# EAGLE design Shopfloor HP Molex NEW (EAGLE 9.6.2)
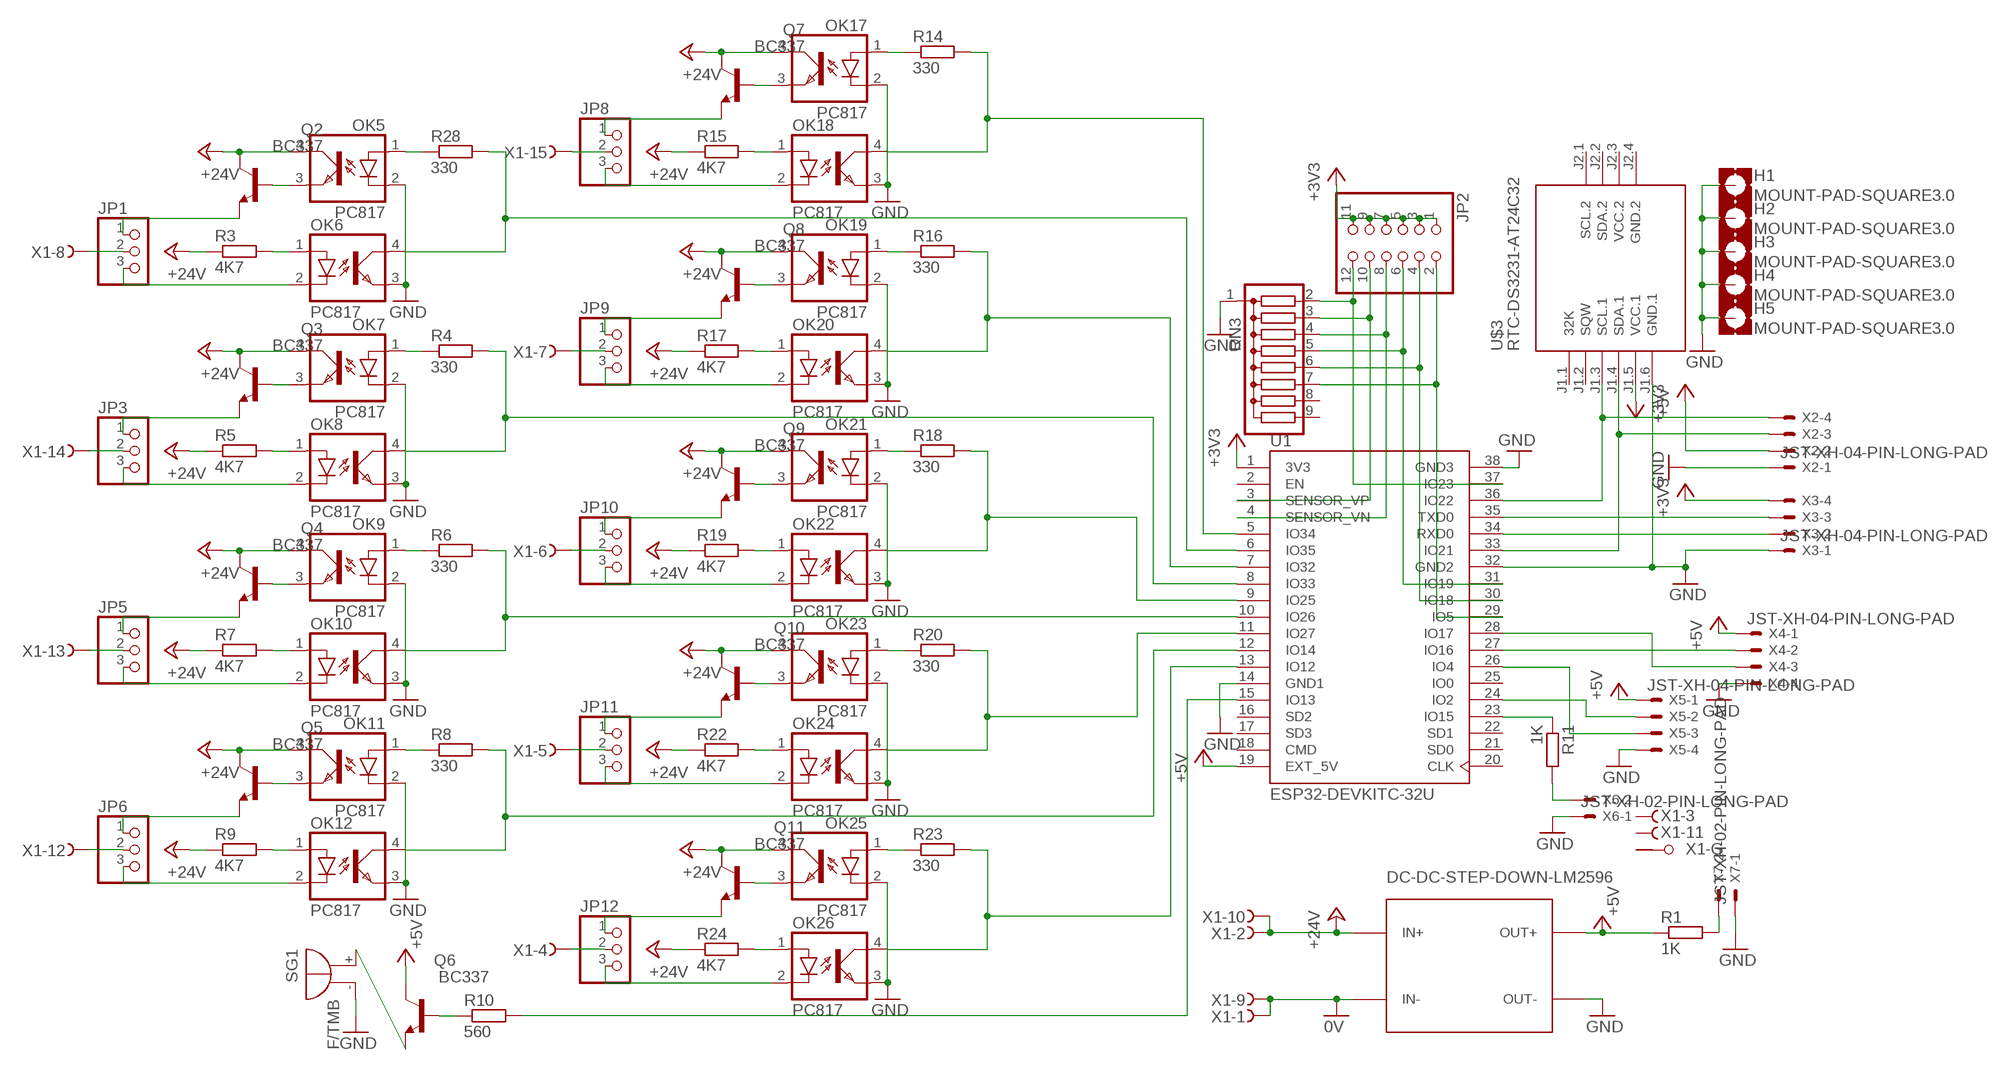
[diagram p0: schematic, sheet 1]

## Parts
H1  MOUNT-PAD-SQUARE3.0  [3,0-PAD-SQUARE]
H2  MOUNT-PAD-SQUARE3.0  [3,0-PAD-SQUARE]
H3  MOUNT-PAD-SQUARE3.0  [3,0-PAD-SQUARE]
H4  MOUNT-PAD-SQUARE3.0  [3,0-PAD-SQUARE]
H5  MOUNT-PAD-SQUARE3.0  [3,0-PAD-SQUARE]
JP1  PINHD-1X3  [1X03]
JP2  PINHD-2X6  [2X06]
JP3  PINHD-1X3  [1X03]
JP5  PINHD-1X3  [1X03]
JP6  PINHD-1X3  [1X03]
JP8  PINHD-1X3  [1X03]
JP9  PINHD-1X3  [1X03]
JP10  PINHD-1X3  [1X03]
JP11  PINHD-1X3  [1X03]
JP12  PINHD-1X3  [1X03]
OK5  PC817  [DIL04]
OK6  PC817  [DIL04]
OK7  PC817  [DIL04]
OK8  PC817  [DIL04]
OK9  PC817  [DIL04]
OK10  PC817  [DIL04]
OK11  PC817  [DIL04]
OK12  PC817  [DIL04]
OK17  PC817  [DIL04]
OK18  PC817  [DIL04]
OK19  PC817  [DIL04]
OK20  PC817  [DIL04]
OK21  PC817  [DIL04]
OK22  PC817  [DIL04]
OK23  PC817  [DIL04]
OK24  PC817  [DIL04]
OK25  PC817  [DIL04]
OK26  PC817  [DIL04]
Q2  BC337  [TO92]
Q3  BC337  [TO92]
Q4  BC337  [TO92]
Q5  BC337  [TO92]
Q6  BC337  [TO92]
Q7  BC337  [TO92]
Q8  BC337  [TO92]
Q9  BC337  [TO92]
Q10  BC337  [TO92]
Q11  BC337  [TO92]
R1  1K  R-EU_0207/7  [0207/7]
R3  4K7  R-EU_0207/7  [0207/7]
R4  330  R-EU_0207/7  [0207/7]
R5  4K7  R-EU_0207/7  [0207/7]
R6  330  R-EU_0207/7  [0207/7]
R7  4K7  R-EU_0207/7  [0207/7]
R8  330  R-EU_0207/7  [0207/7]
R9  4K7  R-EU_0207/7  [0207/7]
R10  560  R-EU_0207/7  [0207/7]
R11  1K  R-EU_0207/7  [0207/7]
R14  330  R-EU_0207/7  [0207/7]
R15  4K7  R-EU_0207/7  [0207/7]
R16  330  R-EU_0207/7  [0207/7]
R17  4K7  R-EU_0207/7  [0207/7]
R18  330  R-EU_0207/7  [0207/7]
R19  4K7  R-EU_0207/7  [0207/7]
R20  330  R-EU_0207/7  [0207/7]
R22  4K7  R-EU_0207/7  [0207/7]
R23  330  R-EU_0207/7  [0207/7]
R24  4K7  R-EU_0207/7  [0207/7]
R28  330  R-EU_0207/7  [0207/7]
RN3  G08R  [SIL9]
SG1  F/TMB  [F/TMB]
U1  ESP32-DEVKITC-32U  [MODULE_ESP32-DEVKITC-32U]
U$1  DC-DC-STEP-DOWN-LM2596  [DC-DC-STEP-DOWN-LM2596]
U$3  RTC-DS3231-AT24C32  [RTC-DS3231-AT24C32]
X1  F15HPS  [F15HP]
X2  JST-XH-04-PIN-LONG-PAD  [JST-XH-04-PACKAGE-LONG-PAD]
X3  JST-XH-04-PIN-LONG-PAD  [JST-XH-04-PACKAGE-LONG-PAD]
X4  JST-XH-04-PIN-LONG-PAD  [JST-XH-04-PACKAGE-LONG-PAD]
X5  JST-XH-04-PIN-LONG-PAD  [JST-XH-04-PACKAGE-LONG-PAD]
X6  JST-XH-02-PIN-LONG-PAD  [JST-XH-02-PACKAGE-LONG-PAD]
X7  JST-XH-02-PIN-LONG-PAD  [JST-XH-02-PACKAGE-LONG-PAD]

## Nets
0V: U$1.IN- X1.1(-1:F) X1.9(-9:F)
+3V3: JP2.1 JP2.3 JP2.5 JP2.7 JP2.9 JP2.11 U1.1(3V3) U$3.J1.5(VCC.1) X3.4
+5V: Q6.3(C) R1.1 U1.19(EXT_5V) U$1.OUT+ X2.2 X4.1 X5.1
+24V: OK5.4(COL) OK7.4(COL) OK9.4(COL) OK11.4(COL) OK17.4(COL) OK19.4(COL) OK21.4(COL) OK23.4(COL) OK25.4(COL) Q2.3(C) Q3.3(C) Q4.3(C) Q5.3(C) Q7.3(C) Q8.3(C) Q9.3(C) Q10.3(C) Q11.3(C) R3.1 R5.1 R7.1 R9.1 R15.1 R17.1 R19.1 R22.1 R24.1 U$1.IN+ X1.2(-2:F) X1.10(-10:F)
GND: H1.B3,0(MOUNT) H2.B3,0(MOUNT) H3.B3,0(MOUNT) H4.B3,0(MOUNT) H5.B3,0(MOUNT) OK5.2(C) OK6.3(EMIT) OK7.2(C) OK8.3(EMIT) OK9.2(C) OK10.3(EMIT) OK11.2(C) OK12.3(EMIT) OK17.2(C) OK18.3(EMIT) OK19.2(C) OK20.3(EMIT) OK21.2(C) OK22.3(EMIT) OK23.2(C) OK24.3(EMIT) OK25.2(C) OK26.3(EMIT) RN3.1 SG1.- U1.14(GND1) U1.32(GND2) U1.38(GND3) U$1.OUT- U$3.J1.6(GND.1) X2.1 X3.1 X4.4 X5.4 X6.1 X7.1
N$1: U1.35(TXD0) X3.3
N$2: JP2.12 RN3.2 U1.37(IO23)
N$3: R11.2 X6.2
N$4: JP1.2 X1.8(-8:F)
N$5: U1.27(IO16) X4.2
N$6: JP2.10 RN3.3 U1.3(SENSOR_VP)
N$7: JP2.8 RN3.4 U1.4(SENSOR_VN)
N$8: JP2.6 RN3.5 U1.31(IO19)
N$9: U1.26(IO4) X5.3
N$10: U1.24(IO2) X5.2
N$11: R11.1 U1.23(IO15)
N$12: Q6.2(B) R10.1
N$13: JP2.4 RN3.6 U1.30(IO18)
N$14: Q6.1(E) SG1.+
N$15: JP8.2 X1.15(-15:F)
N$16: R1.2 X7.2
N$17: JP2.2 RN3.7 U1.29(IO5)
N$19: OK6.4(COL) R28.2 U1.6(IO35)
N$20: OK20.4(COL) R16.2 U1.7(IO32)
N$21: OK8.4(COL) R4.2 U1.8(IO33)
N$22: OK22.4(COL) R18.2 U1.9(IO25)
N$23: OK10.4(COL) R6.2 U1.10(IO26)
N$24: OK24.4(COL) R20.2 U1.11(IO27)
N$25: U1.28(IO17) X4.3
N$26: OK12.4(COL) R8.2 U1.12(IO14)
N$27: U1.33(IO21) U$3.J1.4(SDA.1) X2.3
N$28: OK26.4(COL) R23.2 U1.13(IO12)
N$29: U1.36(IO22) U$3.J1.3(SCL.1) X2.4
N$30: R10.2 U1.15(IO13)
N$31: OK5.1(A) R28.1
N$32: OK5.3(EMIT) Q2.2(B)
N$33: OK6.1(A) R3.2
N$34: JP1.1 Q2.1(E)
N$35: JP1.3 OK6.2(C)
N$36: JP9.2 X1.7(-7:F)
N$37: OK7.1(A) R4.1
N$38: OK7.3(EMIT) Q3.2(B)
N$39: OK8.1(A) R5.2
N$40: JP3.1 Q3.1(E)
N$41: JP3.3 OK8.2(C)
N$42: JP10.2 X1.6(-6:F)
N$43: OK9.1(A) R6.1
N$44: OK9.3(EMIT) Q4.2(B)
N$45: OK10.1(A) R7.2
N$46: U1.34(RXD0) X3.2
N$47: JP5.1 Q4.1(E)
N$48: JP5.3 OK10.2(C)
N$49: JP11.2 X1.5(-5:F)
N$50: OK11.1(A) R8.1
N$51: OK11.3(EMIT) Q5.2(B)
N$52: OK12.1(A) R9.2
N$53: JP6.1 Q5.1(E)
N$54: JP6.3 OK12.2(C)
N$55: OK18.4(COL) R14.2 U1.5(IO34)
N$56: JP12.2 X1.4(-4:F)
N$63: OK17.1(A) R14.1
N$64: OK17.3(EMIT) Q7.2(B)
N$65: OK18.1(A) R15.2
N$66: JP8.1 Q7.1(E)
N$68: JP8.3 OK18.2(C)
N$69: JP6.2 X1.12(-12:F)
N$70: OK19.1(A) R16.1
N$71: OK19.3(EMIT) Q8.2(B)
N$72: OK20.1(A) R17.2
N$73: JP9.1 Q8.1(E)
N$74: JP9.3 OK20.2(C)
N$75: JP5.2 X1.13(-13:F)
N$76: OK21.1(A) R18.1
N$77: OK21.3(EMIT) Q9.2(B)
N$78: OK22.1(A) R19.2
N$79: JP10.1 Q9.1(E)
N$80: JP10.3 OK22.2(C)
N$81: JP3.2 X1.14(-14:F)
N$82: OK23.1(A) R20.1
N$83: OK23.3(EMIT) Q10.2(B)
N$84: OK24.1(A) R22.2
N$85: JP11.1 Q10.1(E)
N$86: JP11.3 OK24.2(C)
N$88: OK25.1(A) R23.1
N$89: OK25.3(EMIT) Q11.2(B)
N$90: OK26.1(A) R24.2
N$91: JP12.1 Q11.1(E)
N$92: JP12.3 OK26.2(C)
Unconnected: RN3.8 RN3.9 U1.2(EN) U1.16(SD2) U1.17(SD3) U1.18(CMD) U1.20(CLK) U1.21(SD0) U1.22(SD1) U1.25(IO0) U$3.J1.1(32K) U$3.J1.2(SQW) U$3.J2.1(SCL.2) U$3.J2.2(SDA.2) X1.3(-3:F) X1.11(-11:F) X1.G1(-G:G1) X1.G2(-G:G2)

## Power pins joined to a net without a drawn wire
GND.2: U$3.J2.4(GND.2)
VCC.2: U$3.J2.3(VCC.2)

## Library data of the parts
H1-H5 = holes:MOUNT-PAD-SQUARE: MOUNTING PAD, square
JP1 JP3 JP5 JP6 JP8-JP12 = pinhead:PINHD-1X3: PIN HEADER
JP2 = pinhead:PINHD-2X6: PIN HEADER
OK5-OK12 OK17-OK26 = optocoupler:PC817: SHARP OPTO COUPLER; MPN: PC817X4J000F; OC_FARNELL: 9707727; OC_NEWARK: 97K7059
Q2-Q11 = transistor-npn:BC337*: NPN Transistor
R1 R3-R11 R14-R20 R22-R24 R28 = rcl:R-EU_: RESISTOR, European symbol; SPICEPREFIX: R
RN3 = resistor-sil:G08R: SIL RESISTOR; OC_FARNELL: unknown; OC_NEWARK: unknown
SG1 = buzzer:F/TMB: BUZZER; OC_FARNELL: unknown; OC_NEWARK: unknown
U1 = ESP32-DEVKITC-32U:ESP32-DEVKITC-32U: ESP32-DEVKITC Check prices; AVAILABILITY: In Stock; DESCRIPTION: ESP32-WROOM-32UE - Transceiver; 802.11 b/g/n (Wi-Fi, WiFi, WLAN), Bluetooth® Smart Ready 4.x Dual Mode Evaluation Board; MF: Espressif Systems; MP: ESP32-DEVKITC-32U; PACKAGE: None; PRICE: None
U$1 = diy-modules:DC-DC-STEP-DOWN-LM2596: DC/DC Step-Down Regulator based on LM2596-ADJ chip LM2596 datasheet available here: http://www.ti.com/lit/ds/symlink/lm2596.pdf Click here to find device on ebay.com
U$3 = diy-modules-ori:RTC-DS3231-AT24C32: RTC Module with Battery and EEPROM based on DS3231 and AT24C32 chips Tutorial can be found here: https://edwardmallon.wordpress.com/2014/05/21/using-a-cheap-3-ds3231-rtc-at24c32-eeprom-from-ebay/ Click here to find device on ebay.com
X1 = con-subd:F15HPS: SUB-D; OC_FARNELL: unknown; OC_NEWARK: unknown
X2-X5 = Rembrandt Electronics - JST XH Connectors v1-0:JST-XH-04-PIN: JST XH Connector 2 Pin Wire to board connector. Pitch: 2,54 mm, (0.100") Number of pins: 4 Created by Rembrandt Electronics www.rembrandtelectronics.com
X6 X7 = Rembrandt Electronics - JST XH Connectors v1-0:JST-XH-02-PIN: JST XH Connector 2 Pin

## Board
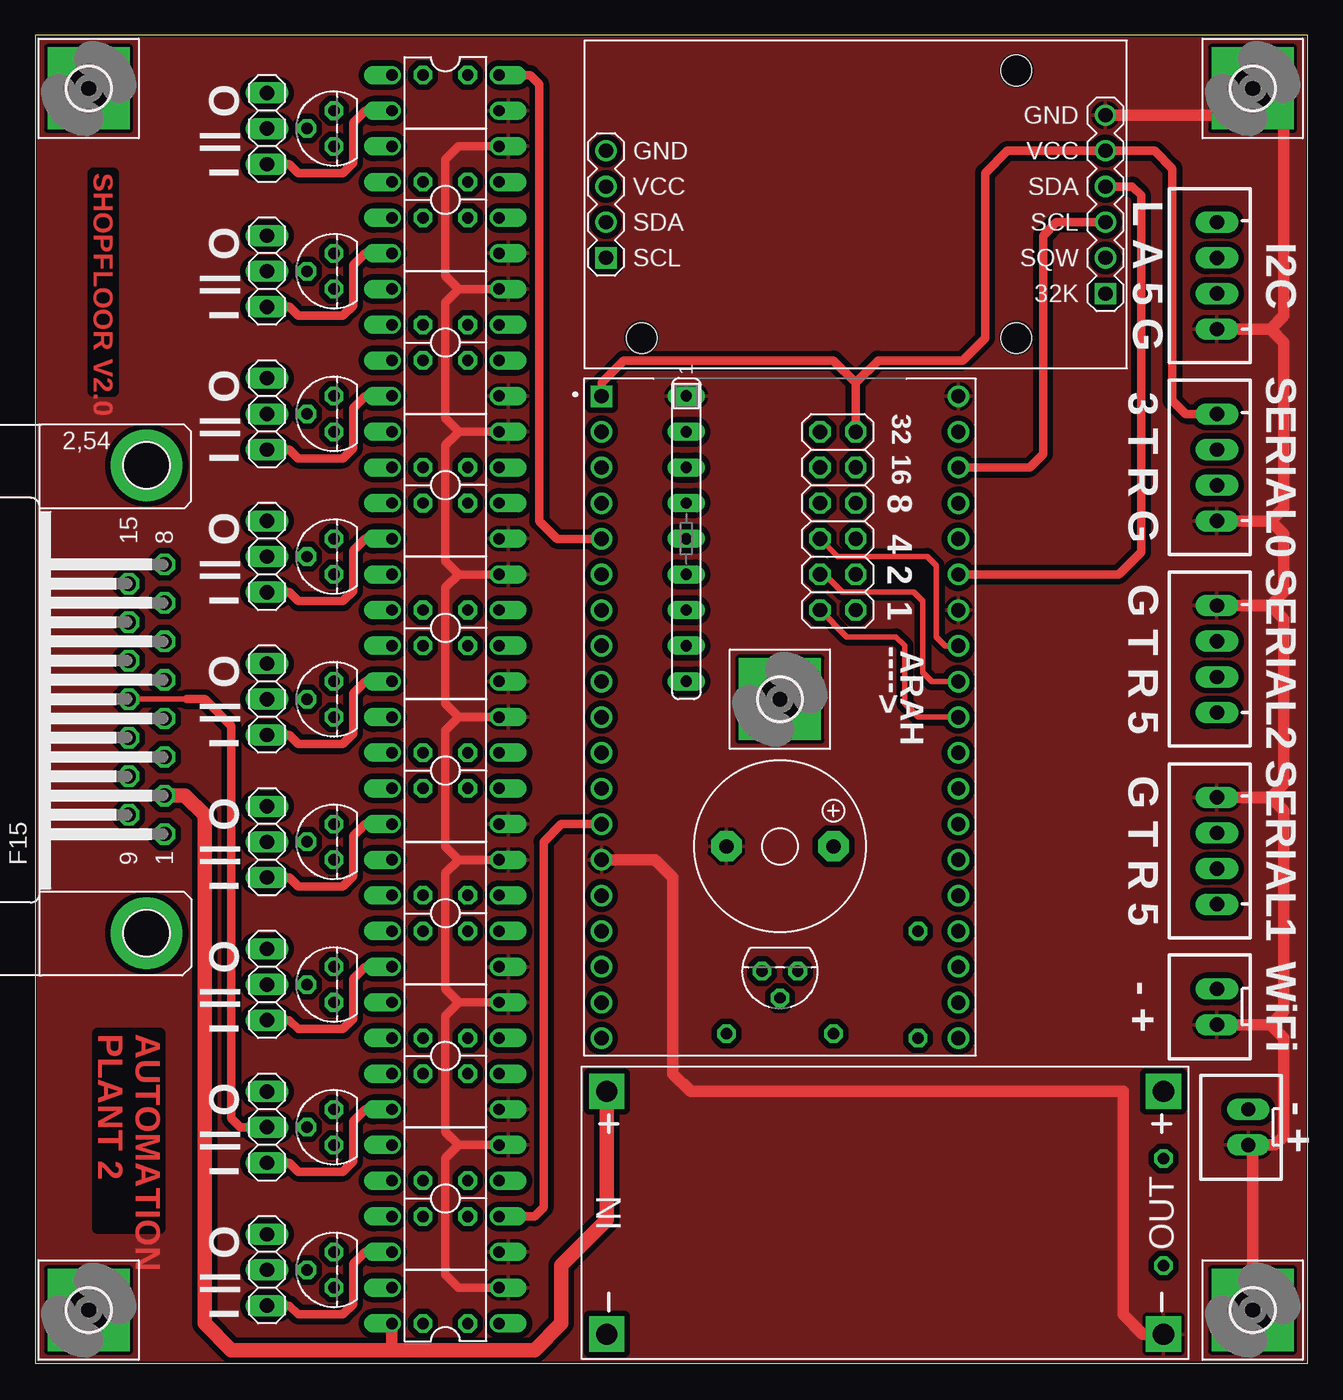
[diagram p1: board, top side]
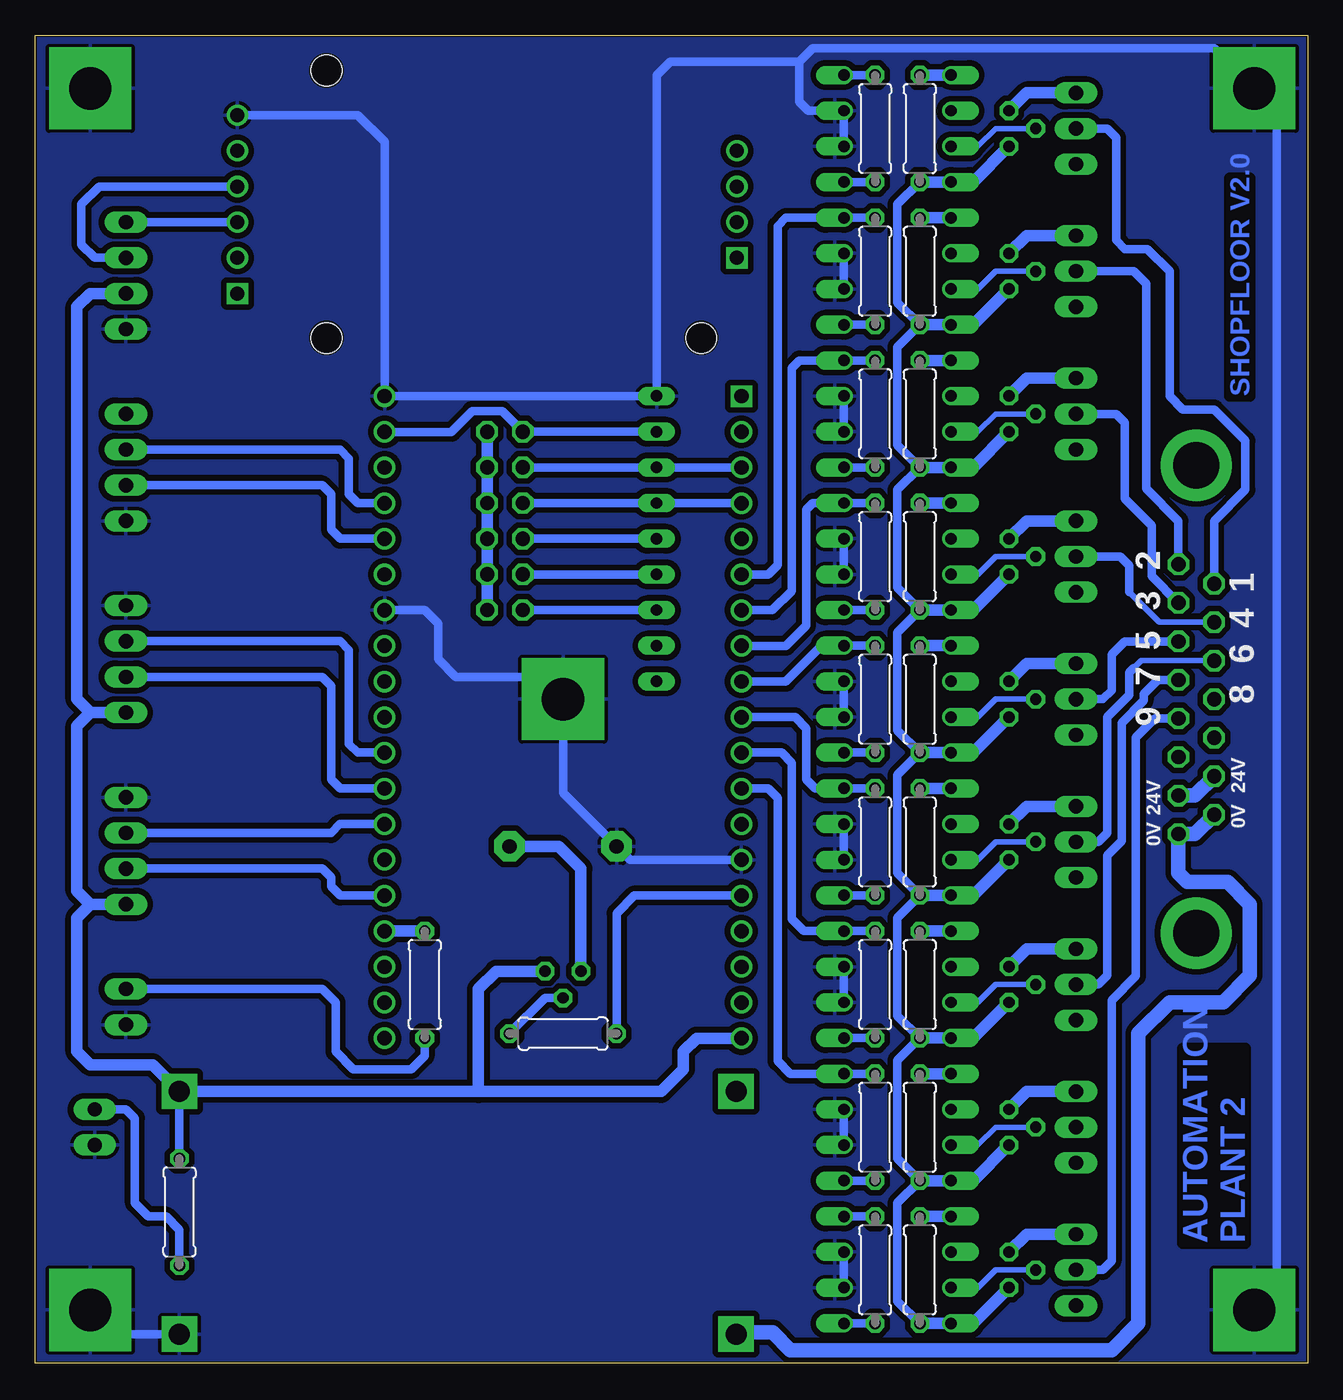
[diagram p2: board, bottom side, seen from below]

Size 90.6 x 94.6 mm. Coordinates in mm from the lower left corner, seen from the top.
Outline: 0,0 90.6,0 90.6,94.6 0,94.6 0,0
Copper layers (1*16): Top 0.035mm / dielectric 1.5mm / Bottom 0.035mm
Design rules "default *": minimum track width 6mil, minimum drill 0.35mm, track to track 16mil, track to pad 16mil, pad to pad 16mil, via to via 16mil, smd to smd 18mil, copper to edge 5mil, drill to drill 6mil, minimum pad ring 10mil, minimum via ring 8mil, stop-mask expansion 4mil, vias tented up to drill 0mil, thermal gap 10mil

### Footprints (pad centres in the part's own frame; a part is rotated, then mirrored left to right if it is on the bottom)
3,0-PAD-SQUARE = drill 3 pad 5.842 square: B3,0 0,0
1X03 = drill 1.016 long: 1 -2.54,0; 2 0,0; 3 2.54,0
2X06 = drill 1.016 octagon: 1 -6.35,-1.27; 2 -6.35,1.27; 3 -3.81,-1.27; 4 -3.81,1.27; 5 -1.27,-1.27; 6 -1.27,1.27; 7 1.27,-1.27; 8 1.27,1.27; 9 3.81,-1.27; 10 3.81,1.27; 11 6.35,-1.27; 12 6.35,1.27
DIL04 = drill 0.813 offset: 1 -1.27,-3.81; 2 1.27,-3.81; 3 1.27,3.81; 4 -1.27,3.81
TO92 = drill 0.813 octagon: 1 1.27,0; 2 0,1.905; 3 -1.27,0
0207/7 = drill 0.813 octagon: 1 -3.81,0; 2 3.81,0
SIL9 = drill 0.813 long: 1 -10.16,0; 2 -7.62,0; 3 -5.08,0; 4 -2.54,0; 5 0,0; 6 2.54,0; 7 5.08,0; 8 7.62,0; 9 10.16,0
F/TMB = drill 1.016 pad 2.159 octagon: + 3.81,0; - -3.81,0
MODULE_ESP32-DEVKITC-32U = drill 1.02 square: 1 -12.7,22.85 | drill 1.02: 2 -12.7,20.31; 3 -12.7,17.77; 4 -12.7,15.23; 5 -12.7,12.69; 6 -12.7,10.15; 7 -12.7,7.61; 8 -12.7,5.07; 9 -12.7,2.53; 10 -12.7,-0.01; 11 -12.7,-2.55; 12 -12.7,-5.09; 13 -12.7,-7.63; 14 -12.7,-10.17; 15 -12.7,-12.71; 16 -12.7,-15.25; 17 -12.7,-17.79; 18 -12.7,-20.33; 19 -12.7,-22.87; 20 12.7,-22.87; 21 12.7,-20.33; 22 12.7,-17.79; 23 12.7,-15.25; 24 12.7,-12.71; 25 12.7,-10.17; 26 12.7,-7.63; 27 12.7,-5.09; 28 12.7,-2.55; 29 12.7,-0.01; 30 12.7,2.53; 31 12.7,5.07; 32 12.7,7.61; 33 12.7,10.15; 34 12.7,12.69; 35 12.7,15.23; 36 12.7,17.77; 37 12.7,20.31; 38 12.7,22.85
DC-DC-STEP-DOWN-LM2596 = drill 1.5 pad 2.5 square: IN+ -19.812,8.636; IN- -19.812,-8.636; OUT+ 19.812,8.636; OUT- 19.812,-8.636
RTC-DS3231-AT24C32 = drill 1 square: J1.1 -17.78,6.35; J2.1 17.78,3.81 | drill 1: J1.2 -17.78,3.81; J1.3 -17.78,1.27; J1.4 -17.78,-1.27; J1.5 -17.78,-3.81; J1.6 -17.78,-6.35; J2.2 17.78,1.27; J2.3 17.78,-1.27; J2.4 17.78,-3.81 | hole 2.2: -11.43,-9.525; -11.43,9.525; 15.24,9.525
F15HP = drill 1.016 octagon: 1 -9.601,-1.27; 2 -6.858,-1.27; 3 -4.115,-1.27; 4 -1.372,-1.27; 5 1.372,-1.27; 6 4.115,-1.27; 7 6.858,-1.27; 8 9.601,-1.27; 9 -8.23,1.27; 10 -5.486,1.27; 11 -2.743,1.27; 12 0,1.27; 13 2.743,1.27; 14 5.486,1.27; 15 8.23,1.27 | drill 3.302 pad 5.08: G1 -16.662,0; G2 16.662,0
JST-XH-04-PACKAGE-LONG-PAD = drill 1.016 long: 1 -3.81,0; 2 -1.27,0; 3 1.27,0; 4 3.81,0
JST-XH-02-PACKAGE-LONG-PAD = drill 1.016 long: 1 -1.27,0; 2 1.27,0

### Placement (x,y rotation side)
H1  3.81,3.81 0 top
H2  3.81,90.81 0 top
H3  53.02,47.31 0 top
H4  86.68,3.81 0 top
H5  86.68,90.81 0 top
JP1  16.51,77.79 270 top
JP2  57.15,60.01 90 top
JP3  16.51,57.47 270 top
JP5  16.51,37.15 270 top
JP6  16.51,16.83 270 top
JP8  16.51,87.95 270 top
JP9  16.51,67.63 270 top
JP10  16.51,47.31 270 top
JP11  16.51,26.99 270 top
JP12  16.51,6.67 270 top
OK5  29.21,75.25 90 top
OK6  29.21,80.33 270 top
OK7  29.21,54.93 90 top
OK8  29.21,60.01 270 top
OK9  29.21,34.61 90 top
OK10  29.21,39.69 270 top
OK11  29.21,14.29 90 top
OK12  29.21,19.37 270 top
OK17  29.21,85.41 90 top
OK18  29.21,90.49 270 top
OK19  29.21,65.09 90 top
OK20  29.21,70.17 270 top
OK21  29.21,44.77 90 top
OK22  29.21,49.85 270 top
OK23  29.21,24.45 90 top
OK24  29.21,29.53 270 top
OK25  29.21,4.13 90 top
OK26  29.21,9.21 270 top
Q2  21.27,77.79 90 top
Q3  21.27,57.47 90 top
Q4  21.27,37.15 90 top
Q5  21.27,16.83 90 top
Q6  53.02,27.94 180 top
Q7  21.27,87.95 90 top
Q8  21.27,67.63 90 top
Q9  21.27,47.31 90 top
Q10  21.27,26.99 90 top
Q11  21.27,6.67 90 top
R1  80.33,10.79 270 bottom
R3  27.62,77.79 90 bottom
R4  30.8,57.47 90 bottom
R5  27.62,57.47 90 bottom
R6  30.8,37.15 90 bottom
R7  27.62,37.15 90 bottom
R8  30.8,16.83 90 bottom
R9  27.62,16.83 90 bottom
R10  53.02,23.5 0 bottom
R11  62.87,26.99 270 bottom
R14  30.8,87.95 90 bottom
R15  27.62,87.95 90 bottom
R16  30.8,67.63 90 bottom
R17  27.62,67.63 90 bottom
R18  30.8,47.31 90 bottom
R19  27.62,47.31 90 bottom
R20  30.8,26.99 90 bottom
R22  27.62,26.99 90 bottom
R23  30.8,6.67 90 bottom
R24  27.62,6.67 90 bottom
R28  30.8,77.79 90 bottom
RN3  46.35,58.74 270 top
SG1  53.02,36.83 0 top
U1  53.02,46.04 0 top
U$1  60.52,10.73 0 top
U$3  58.42,82.55 180 top
X1  7.94,47.31 90 top
X2  84.14,77.47 90 top
X3  84.14,63.82 90 top
X4  84.14,50.16 90 top
X5  84.14,36.51 90 top
X6  84.14,25.4 90 top
X7  86.36,16.83 90 top

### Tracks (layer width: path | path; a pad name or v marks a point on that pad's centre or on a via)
0V
  Bottom 1.016: X1.9 8.04,37.71 X1.1 9.21,34.92 8.57,34.29 5.71,34.29 4.13,32.7 4.13,27.62 6.03,25.72 9.84,25.72 12.06,23.5 12.06,2.86 13.97,0.95 36.83,0.95 38.1,2.22 40.58,2.22 U$1.IN-
+3V3
  Top 0.61: U1.1 40.32,69.85 41.91,71.44 56.83,71.44 58.42,69.85 | JP2.11 58.42,69.85 | 58.42,69.85 60.01,71.44 66.04,71.44 67.63,73.03 67.63,84.77 69.22,86.36 U$3.J1.5 79.69,86.36 80.96,85.09 80.96,68.58 81.92,67.63 X3.4
  Bottom 0.813: JP2.11 JP2.9 JP2.7 JP2.5 JP2.3 JP2.1
+5V
  Bottom 0.61: U$1.OUT+ R1.1
  Bottom 0.813: U1.19 43.51,23.17 44.45,22.23 44.45,20.95 46.04,19.37 59.05,19.37 | 59.05,19.37 U$1.OUT+ 82.23,21.27 86.68,21.27 87.63,22.23 87.63,31.75 86.68,32.7 | Q6.3 57.78,27.94 59.05,26.67 59.05,19.37 | X5.1 86.68,32.7 | 86.68,32.7 87.63,33.66 87.63,45.4 86.68,46.35 | X4.1 86.68,46.35 | 86.68,46.35 87.63,47.31 87.63,75.25 86.68,76.2 X2.2
+24V
  Top 0.813: OK25.4 25.4,0.95
  Top 1.016: X1.2 10.67,40.45 12.06,39.05 12.06,2.86 13.97,0.95 25.4,0.95 35.56,0.95 37.47,2.86 37.47,6.99 40.7,10.22 U$1.IN+
  Bottom 0.61: R15.1 29.21,82.55 29.21,75.56 R3.1 29.21,72.39 29.21,65.41 R17.1 29.21,62.23 29.21,55.24 R5.1 29.21,52.07 29.21,45.09 R19.1 29.21,41.91 29.21,34.92 R7.1 29.21,31.75 29.21,24.77 R22.1 29.21,21.59 29.21,14.61 R9.1 29.21,11.43 29.21,4.45 R24.1
  Bottom 0.813: R24.1 OK25.4 23.81,2.86 Q11.3 | R9.1 OK11.4 23.81,13.02 Q5.3 | R22.1 OK23.4 23.81,23.18 Q10.3 | R7.1 OK9.4 23.81,33.34 Q4.3 | R19.1 OK21.4 23.81,43.5 Q9.3 | R5.1 OK7.4 23.81,53.66 Q3.3 | R17.1 OK19.4 23.81,63.82 Q8.3 | R3.1 OK5.4 23.81,73.98 Q2.3 | R15.1 OK17.4 23.81,84.14 Q7.3
  Bottom 1.016: X1.10 8.04,40.45 X1.2
GND
  Top 0.61: OK17.2 30.16,86.68 29.21,85.72 29.21,77.47 30.16,76.52 | OK5.2 30.16,76.52 | 30.16,76.52 29.21,75.56 29.21,67.31 30,66.52 | 30,66.52 30.16,66.36 OK19.2 | 30,66.52 30,66.2 29.21,65.41 29.21,57.15 30.16,56.2 | OK7.2 30.16,56.2 | 30.16,56.2 29.21,55.24 29.21,46.99 30.16,46.04 | OK21.2 30.16,46.04 | 30.16,46.04 29.21,45.09 29.21,36.83 30.16,35.88 | OK9.2 30.16,35.88 | 30.16,35.88 29.21,34.92 29.21,26.67 30.16,25.72 | OK23.2 30.16,25.72 | 30.16,25.72 29.21,24.77 29.21,16.51 30.16,15.56 | OK11.2 30.16,15.56 | 30.16,15.56 29.21,14.61 29.21,6.35 30.16,5.4 OK25.2
  Top 0.813: U$1.OUT- 78.87,2.1 77.47,3.49 77.47,19.37 46.67,19.37 45.4,20.64 45.4,34.61 44.14,35.87 U1.14 | H4.B3,0 86.68,15.24 X7.1 88.27,15.56 88.9,16.19 88.9,23.18 87.95,24.13 | 87.95,24.13 X6.1 | 87.95,24.13 88.9,25.08 88.9,39.37 87.95,40.32 | 87.95,53.98 88.9,53.02 88.9,41.27 87.95,40.32 | X4.4 87.95,53.98 | 87.95,53.98 88.9,54.93 88.9,59.05 87.95,60.01 | X3.1 87.95,60.01 | 87.95,60.01 88.9,60.96 88.9,72.71 87.95,73.66 | X2.1 87.95,73.66 | 87.95,73.66 88.9,74.61 88.9,89.53 87.63,90.81 H5.B3,0 84.77,88.9 U$3.J1.6 | 87.95,40.32 X5.4
  Bottom 0.61: U1.14 48.25,35.87 SG1.- 53.02,40.64 H3.B3,0 54.61,48.9 60.64,48.9 61.91,50.16 61.91,52.7 62.87,53.66 U1.32 | U$3.J1.6 67.63,88.9 65.72,87 U1.38 RN3.1 46.35,91.76 45.4,92.71 36.2,92.71 | H1.B3,0 2.22,5.4 2.22,89.22 H2.B3,0 6.67,93.66 35.24,93.66 36.2,92.71 | OK26.3 OK25.2 | OK11.2 OK12.3 | OK23.2 OK24.3 | OK10.3 OK9.2 | OK22.3 OK21.2 | OK7.2 OK8.3 | OK20.3 OK19.2 | OK17.2 OK18.3 35.56,89.22 36.2,89.85 36.2,92.71 | OK6.3 OK5.2 | U$1.OUT- 84.96,2.1 H4.B3,0
  pour Top: 0,94.61 90.49,94.61 90.49,94.3 90.49,0 89.85,0 0,0
  pour Bottom: 0,94.61 90.49,94.61 90.49,94.3 90.49,0 90.17,0 0,0
N$1
  Bottom 0.61: 65.73,61.28 U1.35 67.62,61.27 68.26,61.91 68.26,64.45 68.9,65.09 X3.3
N$2
  Bottom 0.61: RN3.2 JP2.12 57.35,67.83 59.49,67.83 60.97,66.35 U1.37
N$3
  Bottom 0.61: R11.2 62.87,21.91 63.82,20.95 67.94,20.95 69.22,22.23 69.22,25.72 70.17,26.67 X6.2
N$4
  Bottom 0.61: X1.8 9.21,60.01 11.51,62.31 11.51,76.91 12.38,77.79 JP1.2
N$5
  Bottom 0.61: U1.27 65.73,40.96 68.9,40.96 69.53,41.59 69.53,48.26 70.17,48.9 X4.2
N$6
  Bottom 0.61: JP2.10 RN3.3 46.34,63.81 U1.3
N$7
  Bottom 0.61: U1.4 40.33,61.28 RN3.4 JP2.8
N$8
  Top 0.406: JP2.6 57.15,57.47 63.5,57.47 64.14,56.83 64.14,51.75 64.78,51.11 U1.31
  Bottom 0.61: RN3.5 JP2.6
N$9
  Bottom 0.61: U1.26 68.91,38.41 69.53,37.78 X5.3
N$10
  Bottom 0.61: U1.24 68.89,33.33 69.53,33.97 69.53,34.61 70.17,35.24 X5.2
N$11
  Bottom 0.813: R11.1 U1.23
N$12
  Bottom 0.61: Q6.2 54.29,26.04 R10.1
N$13
  Top 0.406: JP2.4 56.2,56.2 57.47,54.93 62.55,54.93 63.18,54.29 63.18,49.21 63.83,48.57 U1.30
  Bottom 0.61: JP2.4 RN3.6
N$14
  Bottom 0.813: Q6.1 51.75,35.24 53.34,36.83 SG1.+
N$15
  Bottom 0.61: X1.15 6.67,60.01 4.45,62.23 4.45,65.72 6.67,67.94 8.89,67.94 9.84,68.9 9.84,77.79 11.43,79.38 13.02,79.38 13.65,80.01 13.65,87.31 14.29,87.95 JP8.2
N$16
  Bottom 0.61: R1.2 80.33,9.53 81.28,10.48 82.55,10.48 83.5,11.43 83.5,17.46 84.14,18.1 X7.2
N$17
  Top 0.406: JP2.2 57.78,51.75 61.28,51.75 61.91,51.12 61.91,46.99 62.88,46.03 U1.29
  Bottom 0.61: RN3.7 JP2.2
N$19
  Bottom 0.61: U1.6 38.43,56.19 37.74,56.87 37.74,81 37.15,81.6 OK6.4 R28.2
N$20
  Bottom 0.61: U1.7 38.11,53.65 36.73,55.03 36.73,70.9 36.2,71.44 OK20.4 R16.2
N$21
  Bottom 0.61: U1.8 37.16,51.11 35.71,52.55 35.71,60.81 35.24,61.28 OK8.4 R4.2
N$22
  Bottom 0.61: U1.9 37.16,48.57 34.61,51.12 OK22.4 R18.2
N$23
  Bottom 0.61: U1.10 36.5,46.03 35.71,45.24 35.71,41.59 35.08,40.96 OK10.4 R6.2
N$24
  Bottom 0.61: U1.11 37.47,43.5 36.73,42.76 36.73,31.65 35.88,30.8 OK24.4 R20.2
N$25
  Bottom 0.61: U1.28 65.73,43.5 67.63,43.5 68.26,44.13 68.26,50.8 68.9,51.44 X4.3
N$26
  Bottom 0.61: U1.12 38.42,40.96 37.74,40.28 37.74,21.55 36.83,20.64 OK12.4 R8.2
N$27
  Top 0.61: U1.33 77.14,56.19 78.74,57.78 78.74,83.19 78.11,83.82 U$3.J1.4
  Bottom 0.61: U$3.J1.4 86.04,83.82 87.31,82.55 87.31,79.69 86.36,78.74 X2.3
N$28
  Top 0.61: U1.13 37.45,38.41 36.2,37.15 36.2,11.11 35.56,10.48 OK26.4
  Bottom 0.61: R23.2 OK26.4
N$29
  Top 0.61: U1.36 70.79,63.81 71.75,64.77 71.75,80.33 72.71,81.28 U$3.J1.3
  Bottom 0.61: U$3.J1.3 X2.4
N$30
  Bottom 0.61: U1.15 47.95,33.33 49.21,32.07 R10.2
N$31
  Bottom 0.61: R28.1 OK5.1
N$32
  Bottom 0.406: Q2.2 22.23,77.79 23.5,76.52 OK5.3
N$33
  Bottom 0.813: R3.2 OK6.1
N$34
  Bottom 0.813: JP1.1 20,80.33 Q2.1
N$35
  Top 0.61: JP1.3 18.1,75.25 18.73,74.61 21.91,74.61 22.64,75.35 22.64,78.21 23.5,79.06 OK6.2
N$36
  Bottom 0.61: X1.7 11.11,56.07 11.11,59.69 13.02,61.59 13.02,66.99 13.65,67.63 JP9.2
N$37
  Bottom 0.61: R4.1 OK7.1
N$38
  Bottom 0.406: Q3.2 22.23,57.47 23.5,56.2 OK7.3
N$39
  Bottom 0.813: R5.2 OK8.1
N$40
  Bottom 0.813: JP3.1 20,60.01 Q3.1
N$41
  Top 0.61: JP3.3 18.1,54.93 18.73,54.29 21.91,54.29 22.64,55.03 22.64,57.89 23.5,58.74 OK8.2
N$42
  Bottom 0.61: X1.6 13.03,51.42 13.97,50.48 13.97,47.94 14.61,47.31 JP10.2
N$43
  Bottom 0.61: R6.1 OK9.1
N$44
  Bottom 0.406: Q4.2 22.23,37.15 23.5,35.88 OK9.3
N$45
  Bottom 0.813: R7.2 OK10.1
N$46
  Bottom 0.61: U1.34 65.73,58.74 68.9,58.74 69.53,59.37 69.53,61.91 70.17,62.55 X3.2
N$47
  Bottom 0.813: JP5.1 20,39.69 Q4.1
N$48
  Top 0.61: JP5.3 18.1,34.61 18.73,33.97 21.91,33.97 22.64,34.71 22.64,37.57 23.5,38.42 OK10.2
N$49
  Bottom 0.61: X1.5 10.69,48.68 11.68,47.69 11.68,47.2 13.26,45.63 13.26,37.22 14.29,36.2 14.29,35.23 14.28,35.22 14.28,28.92 14.29,28.91 14.29,27.62 14.92,26.99 JP11.2
N$50
  Bottom 0.61: R8.1 OK11.1
N$51
  Bottom 0.406: Q5.2 22.23,16.83 23.5,15.56 OK11.3
N$52
  Bottom 0.813: R9.2 OK12.1
N$53
  Bottom 0.813: JP6.1 20,19.37 Q5.1
N$54
  Top 0.61: JP6.3 18.1,14.29 18.73,13.65 21.91,13.65 22.64,14.39 22.64,17.25 23.5,18.1 OK12.2
N$55
  Top 0.61: U1.5 37.16,58.73 35.88,60.01 35.88,87.31 35.88,88.58 35.88,91.12 35.24,91.76 OK18.4
  Bottom 0.61: R14.2 OK18.4
N$56
  Bottom 0.61: X1.4 10.9,45.94 12.24,44.59 12.24,27.59 13.97,25.87 13.97,7.3 14.61,6.67 JP12.2
N$63
  Bottom 0.61: R14.1 OK17.1
N$64
  Bottom 0.406: Q7.2 22.23,87.95 23.5,86.68 OK17.3
N$65
  Bottom 0.813: R15.2 OK18.1
N$66
  Bottom 0.813: JP8.1 20,90.49 Q7.1
N$68
  Top 0.61: JP8.3 18.1,85.41 18.73,84.77 21.91,84.77 22.64,85.51 22.64,88.37 23.5,89.22 OK18.2
N$69
  Top 0.406: X1.12 10.79,47.31
  Top 0.61: 10.79,47.31 12.06,47.31 13.97,45.4 13.97,17.46 14.61,16.83 JP6.2
N$70
  Bottom 0.61: R16.1 OK19.1
N$71
  Bottom 0.406: Q8.2 22.23,67.63 23.5,66.36 OK19.3
N$72
  Bottom 0.813: R17.2 OK20.1
N$73
  Bottom 0.813: JP9.1 20,70.17 Q8.1
N$74
  Top 0.61: JP9.3 18.1,65.09 18.73,64.45 21.91,64.45 22.64,65.19 22.64,68.05 23.5,68.9 OK20.2
N$75
  Bottom 0.406: X1.13 11.86,50.05 12.38,49.53
  Bottom 0.61: 12.38,49.53 12.7,49.21 12.7,47.62 14.28,46.05 14.28,44.16 14.29,44.15 14.29,40.31 14.28,40.3 14.28,37.8 14.92,37.15 JP5.2
N$76
  Bottom 0.61: R18.1 OK21.1
N$77
  Bottom 0.406: Q9.2 22.23,47.31 23.5,46.04 OK21.3
N$78
  Bottom 0.813: R19.2 OK22.1
N$79
  Bottom 0.813: JP10.1 20,49.85 Q9.1
N$80
  Top 0.61: JP10.3 18.1,44.77 18.73,44.13 21.91,44.13 22.64,44.87 22.64,47.73 23.5,48.58 OK22.2
N$81
  Bottom 0.406: X1.14 10.57,52.79 12.7,54.93
  Bottom 0.61: JP3.2 13.34,57.47 12.7,56.83 12.7,54.93
N$82
  Bottom 0.61: R20.1 OK23.1
N$83
  Bottom 0.406: Q10.2 22.23,26.99 23.5,25.72 OK23.3
N$84
  Bottom 0.813: R22.2 OK24.1
N$85
  Bottom 0.813: JP11.1 20,29.53 Q10.1
N$86
  Top 0.61: JP11.3 18.1,24.45 18.73,23.81 21.91,23.81 22.64,24.55 22.64,27.41 23.5,28.26 OK24.2
N$88
  Bottom 0.61: R23.1 OK25.1
N$89
  Bottom 0.406: Q11.2 22.23,6.67 23.5,5.4 OK25.3
N$90
  Bottom 0.813: R24.2 OK26.1
N$91
  Bottom 0.813: JP12.1 20,9.21 Q11.1
N$92
  Top 0.61: JP12.3 18.1,4.13 18.73,3.49 21.91,3.49 22.64,4.23 22.64,7.09 23.5,7.94 OK26.2

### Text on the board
Top: SHOPFLOOR V2.0 | AUTOMATION / PLANT 2
Bottom: SHOPFLOOR V2.0 | AUTOMATION / PLANT 2
tNames: O || I | O || I | L A 5 G | I2C | O || I | 32 | 16 | 3 T R G | SERIAL0 | 8 | O || I | 4 | 2 | 1 | ----> | ARAH | O || I | G T R 5 | SERIAL2 | O || I | G T R 5 | SERIAL1 | O || I | - + | WiFi | O || I | - + | O || I
bNames: 2 | 1 | 3 | 4 | 5 | 6 | 7 | 8 | 9 | 24V | 24V | 0V | 0V
_tNames: RN3 | RN3 | X1 | X1 | JP1 | JP1 | J4 | J4 | J6 | J6 | JP2 | JP2 | JP3 | JP3 | SG1 | SG1 | J5 | J5 | U$2 | U$2 | J7 | J7 | X2 | X2 | J8 | J8 | U$1 | U$1 | U1 | U1
_bNames: U$3 | U$3

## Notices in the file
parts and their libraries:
diy-modules: Released under the Creative Commons Attribution 4.0 International License: http://creativecommons.org/licenses/by/4.0
